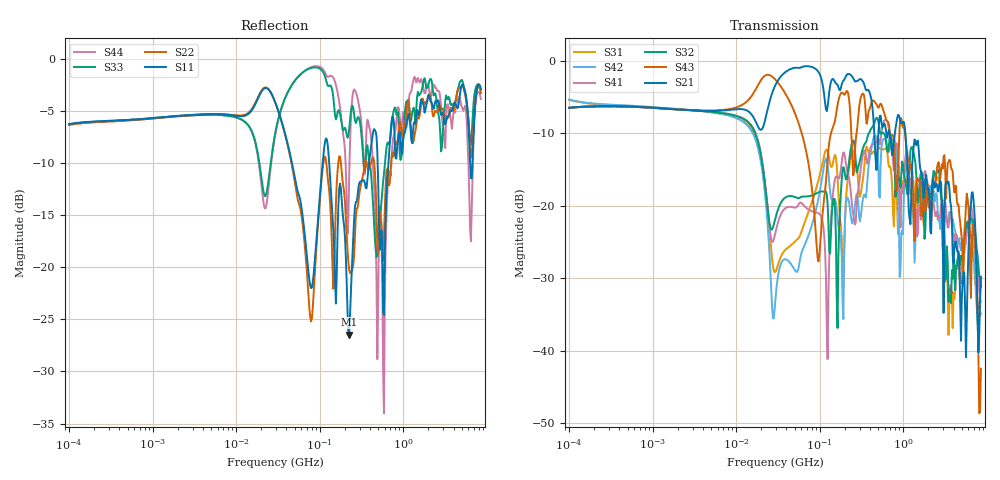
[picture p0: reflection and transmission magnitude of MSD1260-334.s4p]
# MHz S MA R 50
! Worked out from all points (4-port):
!   498 points, 100 kHz to 8.5 GHz, reference 50 ohm
!   strongest paths, dB at 100 kHz, 1.698 MHz, 29.49 MHz, 500.7 MHz, 8.5 GHz:
!     S21: -6.5, -6.7, -3.3, -10.6, -29.8
!     S43: -6.5, -6.7, -2.6, -6.5, -42.5
!     S32: -6.5, -6.6, -21.7, -8.2, -31.2
!     S41: -6.5, -6.7, -23.7, -10.5, -33.2
!     S42: -5.3, -6.6, -32.9, -13.8, -29.8
!     S31: -5.4, -6.6, -29.1, -12.2, -34.9
!   lowest |S11| = -26.5 dB at 225.1 MHz (marker M1), VSWR 1.10, Z = 55 - j0.31 ohm
!   |S11| at or under -10 dB: 129.9 MHz to 388.7 MHz (258.7 MHz wide, 99.8 % of centre); 493.7 MHz to 664.7 MHz (171 MHz wide, 29.5 % of centre); 6.324 GHz to 6.734 GHz (410.1 MHz wide, 6.28 % of centre)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
0.1  0.4873 14.3  0.4746 14.0  0.5371 -13.5  0.473 -166.8
     0.4746 14.0  0.4835 14.3  0.4732 -166.7  0.5407 -13.4
     0.5371 -13.5  0.4732 -166.7  0.4864 14.3  0.4743 13.8
     0.473 -166.8  0.5407 -13.4  0.4743 13.8  0.4837 14.4
13.25948  0.5379 -6.4  0.4562 2.1  0.3694 -90.1  0.388 89.2
          0.4562 2.1  0.5442 -6.8  0.3864 90.0  0.3634 -90.4
          0.3694 -90.1  0.3864 90.0  0.4921 -13.9  0.5209 8.4
          0.388 89.2  0.3634 -90.4  0.5209 8.4  0.4908 -15.0
26.30734  0.6837 -38.4  0.5744 36.6  0.04886 -172.8  0.05832 40.4
          0.5744 36.6  0.6844 -40.7  0.06835 53.8  0.02634 -177.3
          0.04886 -172.8  0.06835 53.8  0.3339 35.5  0.7862 -21.9
          0.05832 40.4  0.02634 -177.3  0.7862 -21.9  0.3191 40.1
96.69917  0.1828 18.3  0.8375 -30.6  0.1503 88.5  0.08877 21.6
          0.8375 -30.6  0.1742 25.6  0.1238 28.2  0.1123 97.1
          0.1503 88.5  0.1238 28.2  0.9055 -25.1  0.04123 -12.5
          0.08877 21.6  0.1123 97.1  0.04123 -12.5  0.9222 -20.2
225.1135  0.04756 -3.4  0.8106 -43.1  0.1833 56.0  0.1537 -4.9
          0.8106 -43.1  0.09764 -33.3  0.2061 50.4  0.1047 17.5
          0.1833 56.0  0.2061 50.4  0.4591 -44.9  0.537 -49.4
          0.1537 -4.9  0.1047 17.5  0.537 -49.4  0.2687 -0.5
2110.57  0.6274 -174.4  0.06631 87.4  0.1241 136.2  0.1255 130.5
         0.06631 87.4  0.6674 -178.4  0.1201 144.9  0.1375 143.2
         0.1241 136.2  0.1201 144.9  0.8021 -178.7  0.09876 18.8
         0.1255 130.5  0.1375 143.2  0.09876 18.8  0.6796 174.8
8500  0.7183 -58.0  0.03239 -53.9  0.01805 -68.0  0.02185 -142.6
      0.03239 -53.9  0.687 -58.0  0.02765 -109.0  0.03219 -65.4
      0.01805 -68.0  0.02765 -109.0  0.7128 -55.2  0.007506 -69.2
      0.02185 -142.6  0.03219 -65.4  0.007506 -69.2  0.6426 -54.4
